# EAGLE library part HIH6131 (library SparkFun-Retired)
Humidity sensor Not in catalog
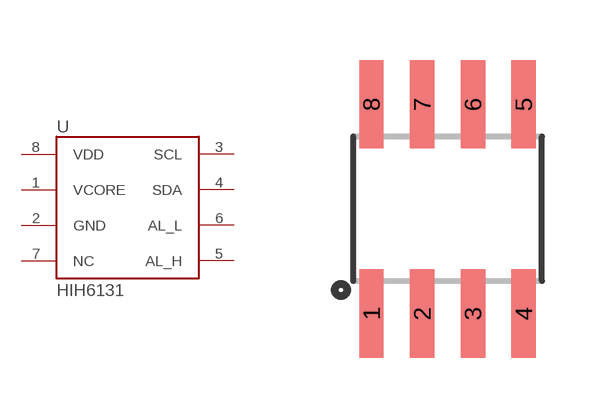
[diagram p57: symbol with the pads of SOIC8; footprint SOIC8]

Designator prefix -

## HIH6131  [SOIC8]
1  VCORE
2  GND
3  SCL
4  SDA
5  AL_H
6  AL_L
7  NC
8  VDD

## Footprint SOIC8 (pad centres in mm)
smd 0.61 x 2.21: 1 -1.905,-2.616; 2 -0.635,-2.616; 3 0.635,-2.616; 4 1.905,-2.616; 5 1.905,2.616; 6 0.635,2.616; 7 -0.635,2.616; 8 -1.905,2.616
